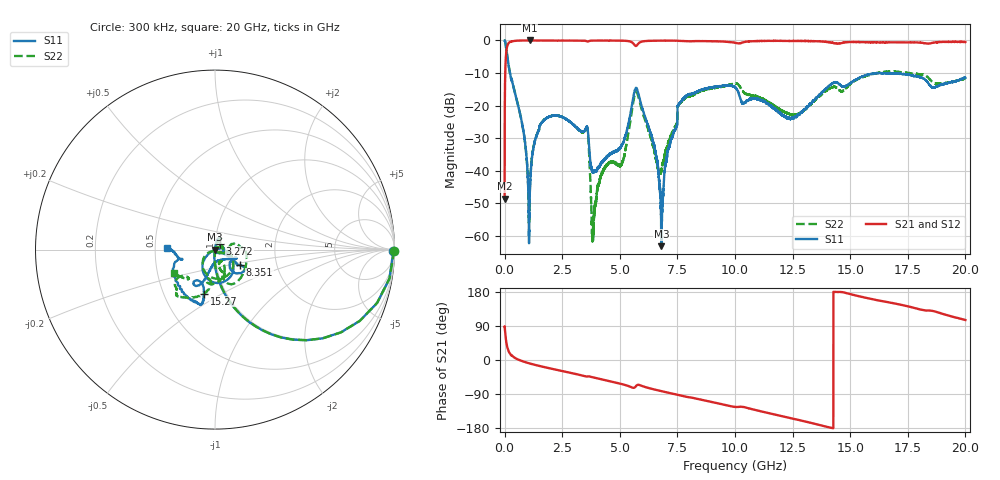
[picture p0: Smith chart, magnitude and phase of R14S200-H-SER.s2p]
!{R14S200}
!Johanson Technology Inc.
!www.johansontechnology.com
!Test Board Conditions:
!Substrate Type  RO4350B
!Substrate Thickness  20 mil
!Substrate Dk  3.66
!TL Type: GCPW
!TL Trace Width  36 mil
!TL Gap  12 mil
!Electrode orientation  Horizontal
!DUT TOPOLOGY	SERIES
!Mounting Pad LxW  26x36 mil
! Created Wed Nov 25 17:33:21 2020
! 2 Port Network Data from SP1.SP block
! freq  magS11  angS11  magS21  angS21  magS12  angS12  magS22  angS22
# khz S ma R 50
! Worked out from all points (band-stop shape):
!   20001 points, 300 kHz to 20 GHz, reference 50 ohm
!   highest |S21| = 0.00 dB at 1.092 GHz (marker M1); lowest = -48.5 dB at 300 kHz (marker M2)
!   |S21| within 3 dB of the highest: 81.3 MHz to end of sweep
!   lowest |S11| = -63.1 dB at 6.804 GHz (marker M3), VSWR 1.00, Z = 50 - j0.0699 ohm
!   |S11| at or under -10 dB: 231 MHz to 16.13 GHz (15.9 GHz wide, 194 % of centre); 16.30582 GHz to 16.36792 GHz (62.11 MHz wide, 0.38 % of centre); 16.37 GHz to end of sweep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
!   |S22| runs from -62.0 to 0.0 dB; largest |S21 - S12| = 0.019
!   S11 on the Smith chart (normalised r, x): 300 kHz: open; 3.272 GHz: 1.05, +0.07; 8.351 GHz: 1.30, -0.23; 15.27 GHz: 0.79, -0.41; 20 GHz: 0.58, +0.01
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300  0.9936 -0.5  0.003742 88.7  0.003755 89.8  0.9983 -0.4
150300  0.4659 -63.3  0.8814 26.7  0.883 26.6  0.4678 -63.2
1092300  0.004259 98.6  0.9999 -9.2  0.9985 -9.2  0.004514 56.2
1281300  0.02513 82.2  0.9983 -12.2  0.9995 -12.2  0.02583 71.8
1661300  0.05757 77.0  0.9976 -17.9  0.9975 -17.8  0.05775 66.7
3272300  0.04171 48.5  0.9958 -39.5  0.9956 -39.4  0.04102 45.2
3334300  0.04 45.5  0.9952 -40.3  0.996 -40.3  0.03941 44.4
3590300  0.04678 -9.2  0.9623 -43.7  0.9622 -43.6  0.04498 -2.5
3854300  0.009723 -34.5  0.9952 -46.1  0.9954 -46.1  0.001331 85.9
4287300  0.01435 -66.6  0.9963 -52.2  0.9968 -52.2  0.01038 159.4
5086300  0.02483 -46.5  0.9919 -63.6  0.9914 -63.6  0.01314 83.9
5702300  0.1873 -79.3  0.8233 -68.9  0.8233 -68.9  0.1643 -75.4
6667300  0.01044 -148.0  0.992 -80.2  0.9915 -80.2  0.009949 -118.7
6804300  0.0006987 -89.1  0.9929 -82.2  0.9923 -82.2  0.009881 -65.5
7600300  0.1103 -29.5  0.986 -93.1  0.986 -93.1  0.1079 17.3
8351300  0.163 -32.0  0.9775 -102.4  0.9776 -102.4  0.1566 2.6
1.00003e7  0.1924 -42.7  0.921 -123.8  0.9214 -123.8  0.2183 -55.3
1.23403e7  0.06507 -69.3  0.9819 -152.6  0.985 -152.5  0.07592 -70.6
1.33343e7  0.1112 -103.4  0.9779 -166.6  0.9797 -166.5  0.108 -61.1
1.52663e7  0.2528 -103.9  0.9465 170.0  0.9519 169.6  0.2476 -103.1
1.66673e7  0.3104 -109.6  0.9358 152.3  0.9272 152.1  0.3335 -128.6
2e7  0.2684 178.0  0.9459 105.5  0.9454 105.6  0.2603 -150.3
